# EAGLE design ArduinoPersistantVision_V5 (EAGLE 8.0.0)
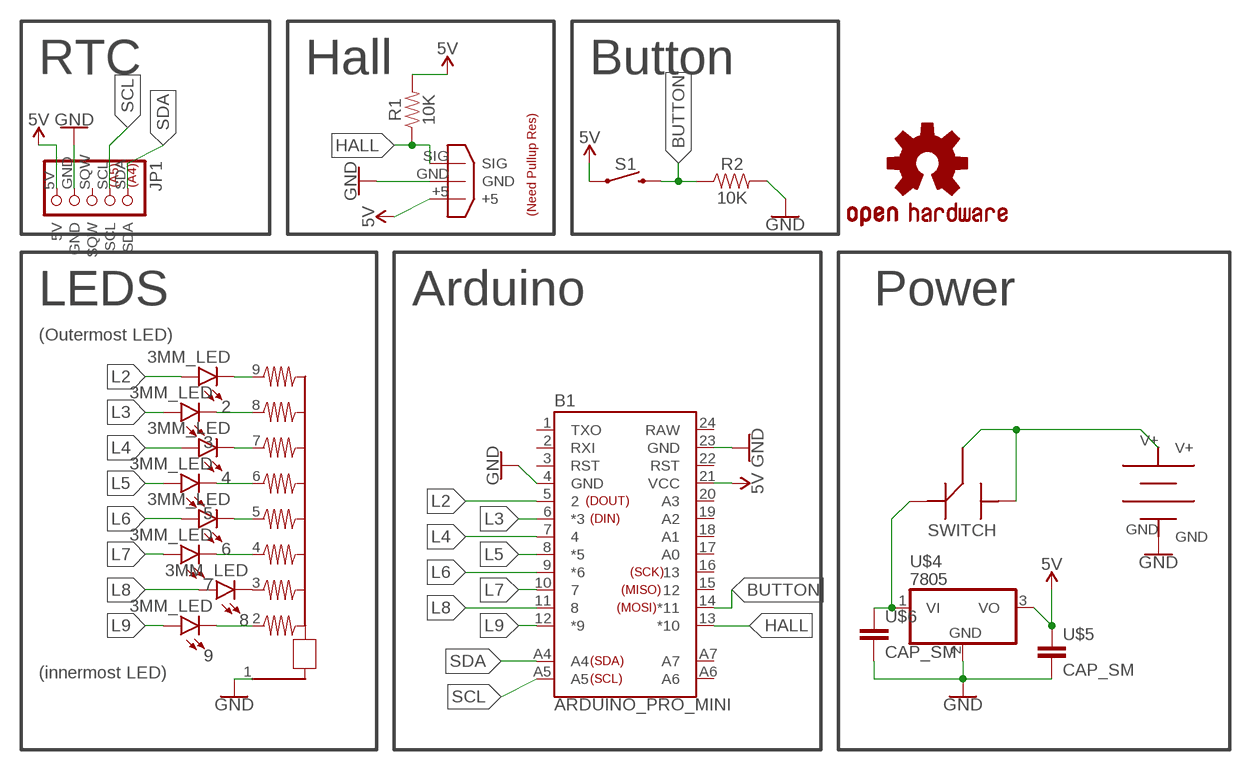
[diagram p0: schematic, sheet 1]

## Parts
2  3MM_LED  [LED_3MM]
3  3MM_LED  [LED_3MM]
4  3MM_LED  [LED_3MM]
5  3MM_LED  [LED_3MM]
6  3MM_LED  [LED_3MM]
7  3MM_LED  [LED_3MM]
8  3MM_LED  [LED_3MM]
9  3MM_LED  [LED_3MM]
B1  ARDUINO_PRO_MINI  [ARDUINO_PRO_MINI]
JP1  SP_RTC  [SP_RTC]
LOGO1  OSHW-LOGOL  [OSHW-LOGO-L]
R1  10K  RES  [AXIAL-0.3]
R2  10K  RES  [AXIAL-0.3]
RN1  RN08  [RN-9]
S1  MOMENTARY-SWITCH-SPST-PTH-6.0MM  [TACTILE_SWITCH_PTH_6.0MM]
SWITCH  RFSWITCH  [RFSWITCH]
U$1  POW  [SCREWTERMINAL-3.5MM-2]
U$2  HALLEFFECT  [HALLSENSOR]
U$4  7805  [TO220V]
U$5  CAP_SM  [CAP_SM]
U$6  CAP_SM  [CAP_SM]

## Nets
5V: B1.21(VCC) JP1.5V R1.P$2 S1.1 U$2.+5 U$4.3(VO) U$5.1
BUTTON: B1.14(*11) R2.P$1 S1.3
GND [POWER]: B1.4(GND) B1.23(GND) JP1.GND R2.P$2 RN1.1 U$1.GND U$2.GND U$4.2(GND) U$5.2 U$6.2
HALL: B1.13(*10) R1.P$1 U$2.SIG
L2: 2.A B1.5
L3: 3.A B1.6(*3)
L4: 4.A B1.7
L5: 5.A B1.8(*5)
L6: 6.A B1.9(*6)
L7: 7.A B1.10
L8: 8.A B1.11
L9: 9.A B1.12(*9)
N$1: SWITCH.P$1 U$4.1(VI) U$6.1
N$2: 9.K(C) RN1.2
N$10: SWITCH.MIDDLE SWITCH.P$2 U$1.V+
N$12: 2.K(C) RN1.9
N$13: 3.K(C) RN1.8
N$14: 4.K(C) RN1.7
N$15: 5.K(C) RN1.6
N$16: 6.K(C) RN1.5
N$17: 7.K(C) RN1.4
N$18: 8.K(C) RN1.3
SCL: B1.A5 JP1.SCL
SDA: B1.A4 JP1.SDA
Unconnected: B1.1(TXO) B1.2(RXI) B1.3(RST) B1.15 B1.16 B1.17(A0) B1.18(A1) B1.19(A2) B1.20(A3) B1.22(RST) B1.A6 B1.A7 JP1.SQW

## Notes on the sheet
- RTC | Hall | Button
- LEDS | Arduino | Power
- (Outermost LED)
- (innermost LED)

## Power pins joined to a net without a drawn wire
RAW: B1.24(RAW)

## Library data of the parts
2-9 = Richard_Components:3MM_LED
B1 = Richard_Micros:ARDUINO_PRO_MINI: SparkFun Pro Mini Pro Mini compatible footprint. Dimensions: 0.7 x 1.3" PCB Thickness: 0.8mm SparkFun Products: 3.3V/8MHz 5V/16MHz
JP1 = Richard_Boards:SP_RTC: PIN HEADER
LOGO1 = SparkFun-Aesthetics:OSHW-LOGO: Open-Source Hardware (OSHW) Logo
R1 R2 = Richard_Components:RES
RN1 = Richard_Components:RN08: RESISTOR NETWORK; OC_FARNELL: unknown; OC_NEWARK: unknown
S1 = Richard:MOMENTARY-SWITCH-SPST: Momentary Switch (Pushbutton) - SPST; PROD_ID: SWCH-08441; SF_SKU: COM-00097
SWITCH = Richard_Components:RFSWITCH
U$1 = Richard:POW
U$2 = Richard:HALLEFFECT
U$4 = Richard_Components:7805
U$5 U$6 = Richard_Components:CAP_SM

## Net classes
0 default: width 0.381 mm
1 POWER: width 0.635 mm

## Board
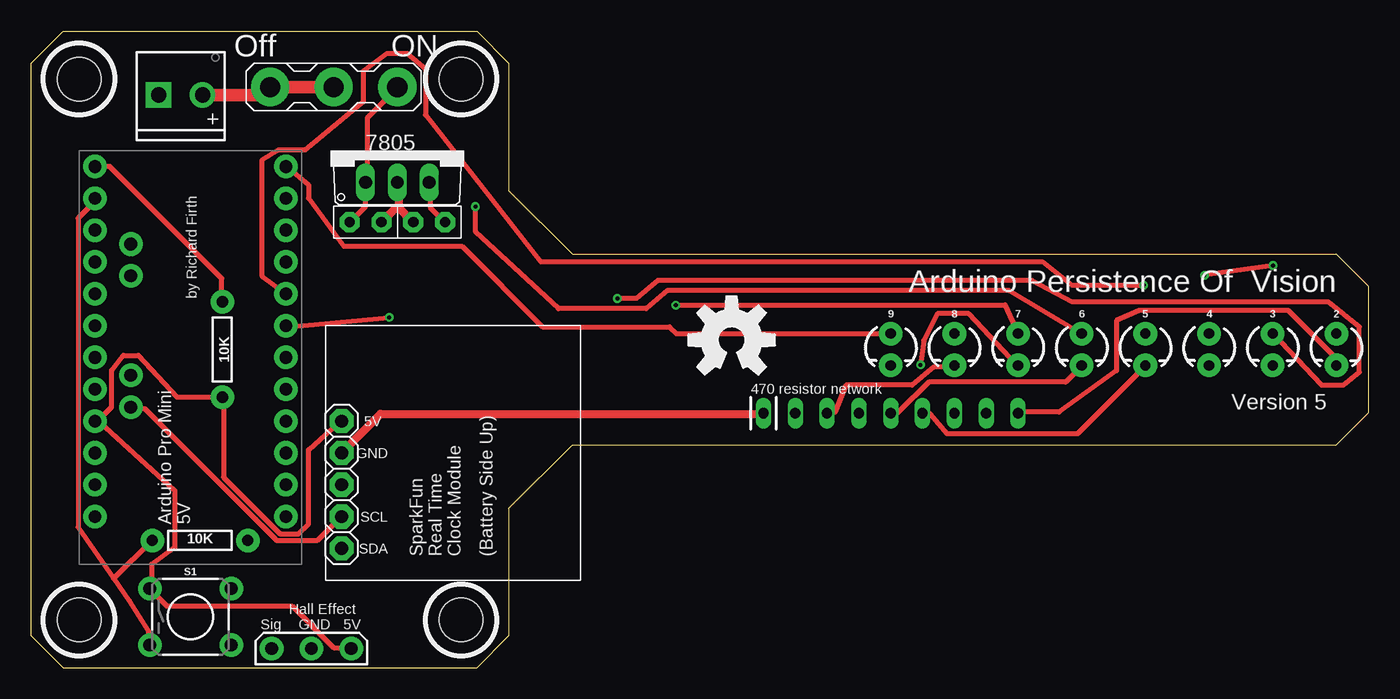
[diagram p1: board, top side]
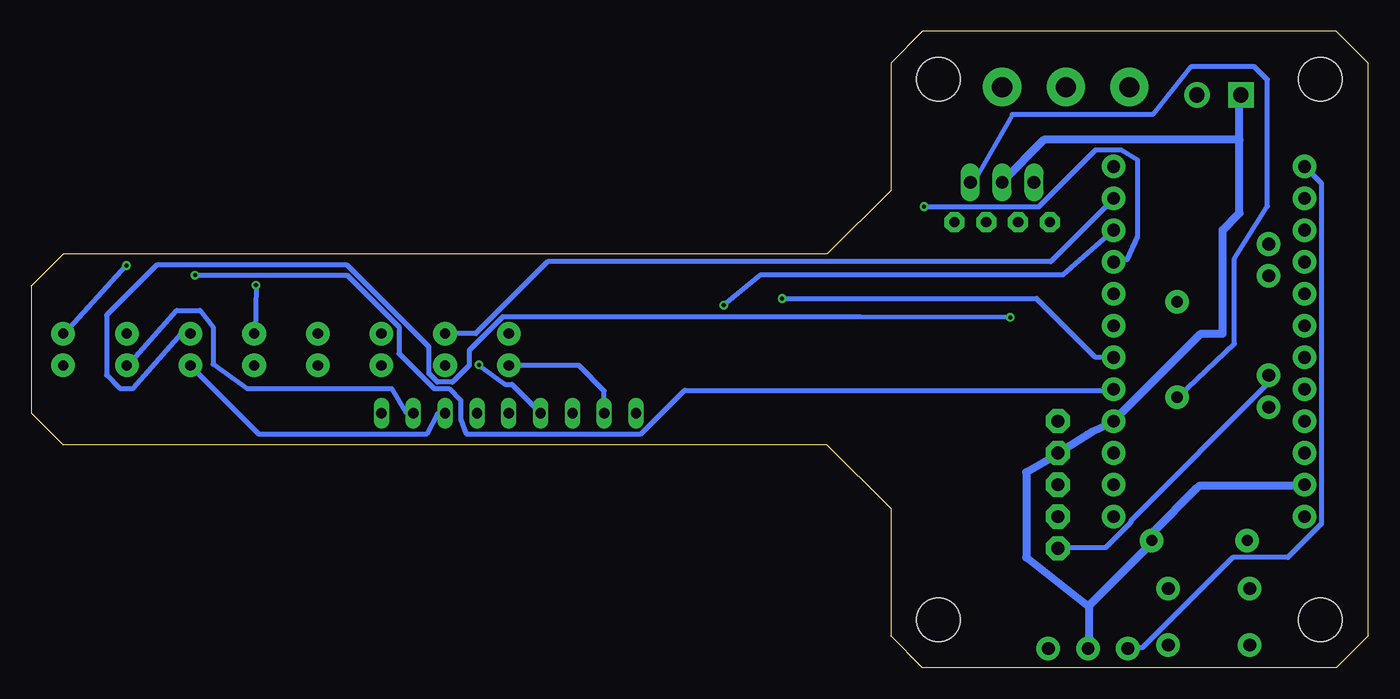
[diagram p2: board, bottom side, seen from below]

Size 106.68 x 50.8 mm. Coordinates in mm from the lower left corner, seen from the top.
Outline: 0,2.54 0,48.26 2.54,50.8 35.56,50.8 38.1,48.26 38.1,38.1 43.18,33.02 104.14,33.02 106.68,30.48 106.68,20.32 104.14,17.78 43.18,17.78 38.1,12.7 38.1,2.54 35.56,0 2.54,0 0,2.54
Copper layers (1*16): Top 0.0356mm / dielectric 1.5011mm / Bottom 0.0356mm
Design rules "LaenPCBOrder": minimum track width 6mil, minimum drill 13mil, track to track 6mil, track to pad 6mil, pad to pad 6mil, via to via 6mil, smd to smd 6mil, copper to edge 15mil, drill to drill 6mil, minimum pad ring 7mil, minimum via ring 7mil, stop-mask expansion 3mil, vias tented up to drill 0mil, thermal gap 10mil
Holes 3.5 mm at 3.81,3.81 34.29,3.81 3.81,46.99 34.29,46.99

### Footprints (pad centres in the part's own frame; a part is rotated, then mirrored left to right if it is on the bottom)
LED_3MM = drill 0.813 pad 1.88: A -1.27,0; K 1.27,0
ARDUINO_PRO_MINI = drill 1.016 pad 1.88: 1 -7.62,12.7; 2 -7.62,10.16; 3 -7.62,7.62; 4 -7.62,5.08; 5 -7.62,2.54; 6 -7.62,0; 7 -7.62,-2.54; 8 -7.62,-5.08; 9 -7.62,-7.62; 10 -7.62,-10.16; 11 -7.62,-12.7; 12 -7.62,-15.24; 13 7.62,-15.24; 14 7.62,-12.7; 15 7.62,-10.16; 16 7.62,-7.62; 17 7.62,-5.08; 18 7.62,-2.54; 19 7.62,0; 20 7.62,2.54; 21 7.62,5.08; 22 7.62,7.62; 23 7.62,10.16; 24 7.62,12.7; A4 4.763,1.429; A5 4.763,3.969; A6 4.763,-9.049; A7 4.763,-6.509
SP_RTC = drill 1.016 pad 1.93 octagon: 5V -5.08,0; GND -2.54,0; SCL 2.54,0; SDA 5.08,0; SQW 0,0
AXIAL-0.3 = drill 0.9 pad 1.88: P$1 -3.81,0; P$2 3.81,0
RN-9 = drill 0.813 long: 1 -10.16,0; 2 -7.62,0; 3 -5.08,0; 4 -2.54,0; 5 0,0; 6 2.54,0; 7 5.08,0; 8 7.62,0; 9 10.16,0
TACTILE_SWITCH_PTH_6.0MM = drill 1.016 pad 1.88: 1 -3.251,2.261; 2 3.251,2.261; 3 -3.251,-2.261; 4 3.251,-2.261
RFSWITCH = drill 1.6 pad 3.048: MIDDLE 0,0; P$1 -5.08,0; P$2 5.08,0
SCREWTERMINAL-3.5MM-2 = drill 1.2 pad 2.032 square: GND 0,0 | drill 1.2 pad 2.032: V+ 3.5,0
HALLSENSOR = drill 1.016 pad 1.88: +5 -3.175,0; GND 0,0; SIG 3.175,0
TO220V = drill 1.016 long: 1 -2.54,-2.54; 2 0,-2.54; 3 2.54,-2.54
CAP_SM = drill 0.813 pad 1.6 octagon: 1 -1.27,0; 2 1.27,0

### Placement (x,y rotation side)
2  104.14,25.4 270 top
3  99.06,25.4 270 top
4  93.98,25.4 270 top
5  88.9,25.4 270 top
6  83.82,25.4 270 top
7  78.74,25.4 270 top
8  73.66,25.4 270 top
9  68.58,25.4 270 top
B1  12.7,24.77 180 top
JP1  24.77,14.61 270 top
LOGO1  55.88,26.16 0 top
R1  15.24,25.4 270 top
R2  13.46,10.16 0 top
RN1  68.58,20.32 0 top
S1  12.7,4.06 0 top
SWITCH  24.13,46.35 180 top
U$1  10.16,45.72 0 top
U$2  22.35,1.52 180 top
U$4  29.21,41.27 0 top
U$5  31.75,35.56 180 top
U$6  26.67,35.56 0 top

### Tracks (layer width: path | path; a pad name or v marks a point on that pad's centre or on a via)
5V
  Top 0.381: U$4.3 31.87,38.67 31.87,36.67 32.94,35.6 U$5.1 | JP1.5V 24.67,19.6 24.42,19.44 22.11,17.39 22.11,11.47 21.31,10.67 19.87,10.67 15.34,15.2 15.34,21.47 R1.P$2 15.2,21.6 11.6,21.6 8.53,24.92 7.33,24.92 6.4,23.74 6.4,20.8 5.33,19.74 B1.21 5.47,19.6 11.44,14.13 11.44,9.6 9.6,8.27 9.6,6.4 S1.1 9.47,6.27 10.8,4.93 20.8,4.93 24.14,1.6 25.47,1.6 U$2.+5
  Bottom 0.381: U$4.3 31.74,38.8 31.47,38.8 28.41,44.15 17.19,44.15 14.13,47.97 9.07,47.97 8.04,46.94 8.04,36.84 10.68,32.67 10.68,25.87 15.2,21.6 R1.P$2
BUTTON
  Top 0.381: 5.2,37.34 B1.14 5.07,37.2 3.73,35.87 3.73,11.2 6.57,7.13 | 6.57,7.13 7.81,5.35 9.34,2.93 S1.3 | R2.P$1 9.6,10.13 6.67,7.2 6.57,7.13
GND
  Top 0.635: 29.34,36.67 29.34,38.67 U$4.2 | 29.34,36.67 30.4,35.6 U$5.2 | U$6.2 28,35.6 29.07,36.67 29.34,36.67 | 22.4,1.6 U$2.GND | RN1.1 58.41,20.27 27.87,20.27 24.8,17.2 JP1.GND
  Bottom 0.635: B1.23 5.2,14.54 13.41,14.54 13.73,14.27 17.2,10.8 17.2,10.27 R2.P$2 17.34,9.87 22.27,4.93 | 10.27,42.14 10.27,36.27 11.6,34.94 11.6,26.67 13.34,26.67 B1.4 20.4,19.6 22.02,18.84 24.67,17.2 JP1.GND 24.94,16.93 27.29,15.6 27.29,8.8 22.54,5.07 22.27,4.93 | 10.27,42.14 10.27,45.61 U$1.GND | 10.27,42.14 25.87,42.14 29.2,38.8 U$4.2 | 22.27,4.93 22.27,1.6 U$2.GND
HALL
  Top 0.381: B1.13 6.27,40.01 15.2,31.07 15.2,29.2 | 15.2,29.08 15.2,29.2 | R1.P$1 15.34,29.2 15.2,29.2
  Bottom 0.381: U$2.SIG 19.07,1.6 18,1.6 10.8,8.8 6.4,8.8 3.73,11.47 3.73,38.67 5.07,40.01 B1.13
L2  (via drill 0.33)
  Top 0.381: v99.09,32.1 v93.62,31.34
  Bottom 0.381: v93.62,31.34 81.48,31.34 77.34,27.2 77.34,25.07 74.54,22.27 73.36,22.27 72.42,21.34 72.42,19.87 71.98,18.67 58.01,18.67 54.54,22.14 20.4,22.14 B1.5 | v99.09,32.1 104.01,26.67 2.A
L3  (via drill 0.33)
  Top 0.381: v46.77,29.47 48.31,29.47 50.01,30.91 79.84,30.91 83.08,29.2 103.48,29.2 105.99,27.2 105.99,23.6 104.68,22.55 102.95,22.55 99.08,26.67 3.A
  Bottom 0.381: v46.77,29.47 26.46,29.47 21.79,24.8 20.4,24.8 B1.6
L4  (via drill 0.33)
  Top 0.381: v28.56,27.96 20.4,27.2 B1.7
  Bottom 0.381: 4.A 94.68,26.67 98.55,22.3 99.61,22.3 100.67,23.35 100.67,28.15 96.68,32.14 81.48,32.14 74.94,25.6 74.94,23.47 74.28,22.8 73.08,22.8 71.74,24.14 71.74,25.34 69.08,28 40.54,28 v28.56,27.96
L5  (via drill 0.33)
  Top 0.381: v88.75,30.54 83.05,30.54 80.68,32.4 40.65,32.4 31.46,44.14 31.46,47.84 30,49.03 28.4,49.03 26.51,47.65 26.51,45.22 21.87,41.34 19.74,41.34 18.43,40.54 18.43,31.2 20.27,29.87 B1.8
  Bottom 0.381: v88.75,30.54 88.81,26.67 5.A
L6  (via drill 0.33)
  Top 0.381: v35.44,36.8 35.45,34.77 42.06,28.67 49.07,28.67 50.78,30.12 78,30.12 83.74,26.67 6.A
  Bottom 0.381: v35.44,36.8 26.27,36.8 21.74,41.34 19.74,41.34 18.43,40.54 18.43,34.4 19.25,32.56 20.27,32.4 B1.9
L7  (via drill 0.33)
  Top 0.381: 7.A 77.7,28.96 74.68,28.94 v51.42,28.94
  Bottom 0.381: v51.42,28.94 48.49,31.36 24.35,31.36 20.4,34.8 B1.10
L8
  Bottom 0.381: B1.11 20.4,37.34 25.34,32.4 65.47,32.4 71.21,26.67 8.A
L9
  Top 0.381: 9.A 51.47,26.67 50.94,27.2 40.8,27.2 34.37,33.64 24.94,33.64 22.11,37.48 22.11,38.55 20.4,40.01 B1.12
N$1
  Top 0.381: U$6.1 25.47,35.6 26.67,36.8 U$4.1 26.8,38.8 26.8,43.87 29.2,46.27 SWITCH.P$1
N$2
  Bottom 0.381: RN1.2 60.96,22.1 62.99,24.13 9.K
N$10
  Top 1.016: SWITCH.MIDDLE SWITCH.P$2 18.41,45.72 U$1.V+
N$12
  Top 0.381: RN1.9 78.81,20.4 82.01,20.4 86.59,23.72 86.59,27.71 88.41,28.51 100.31,28.51 104.01,24.8 104.01,24.14 2.K
N$13
  Bottom 0.381: RN1.8 76.28,20.4 76.81,20.4 77.92,22.27 89.45,22.27 92.17,24.23 92.17,27.2 93.22,28.51 95.08,28.51 98.95,24.14 3.K
N$14
  Bottom 0.381: RN1.7 73.74,20.27 74.28,20.27 75.11,18.67 88.54,18.67 93.88,24 4.K
N$15
  Top 0.381: RN1.6 71.21,20.27 71.74,20.27 73.09,18.67 83.48,18.67 88.81,24 5.K
N$16
  Top 0.381: RN1.5 68.67,20.4 69.21,20.4 71.61,22.8 82.54,22.8 83.74,24 6.K
N$17  (via drill 0.33)
  Top 0.381: v70.95,24.17 71.21,26.14 72.31,28.26 74.81,28.26 78.68,24.14 7.K
  Bottom 0.381: v70.95,24.17 70.94,24.14 68.89,22.61 68.33,22.61 RN1.4
N$18
  Top 0.381: RN1.3 63.61,20.4 64.14,20.4 65.02,22.55 70.3,22.55 72.01,24 73.61,24 8.K
SCL
  Top 0.381: B1.A5 8,20.67 9.07,20.67 19.6,10.13 22.8,10.13 24.67,12 JP1.SCL
SDA
  Bottom 0.381: B1.A4 8,23.34 8,22.67 18.94,11.73 18.94,11.6 20.94,9.6 24.67,9.6 JP1.SDA

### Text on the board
tPlace: Off | ON | Arduino Persistence Of Vision | by Richard Firth | 470 resistor network | Version 5 | 5V | GND | SCL | Arduino Pro Mini / 5V | SDA | SparkFun / Real Time / Clock Module | (Battery Side Up) | Hall Effect | Sig | GND | 5V

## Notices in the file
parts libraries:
SparkFun-PowerSymbols: Licensing: Creative Commons ShareAlike 4.0 International - https://creativecommons.org/licenses/by-sa/4.0
